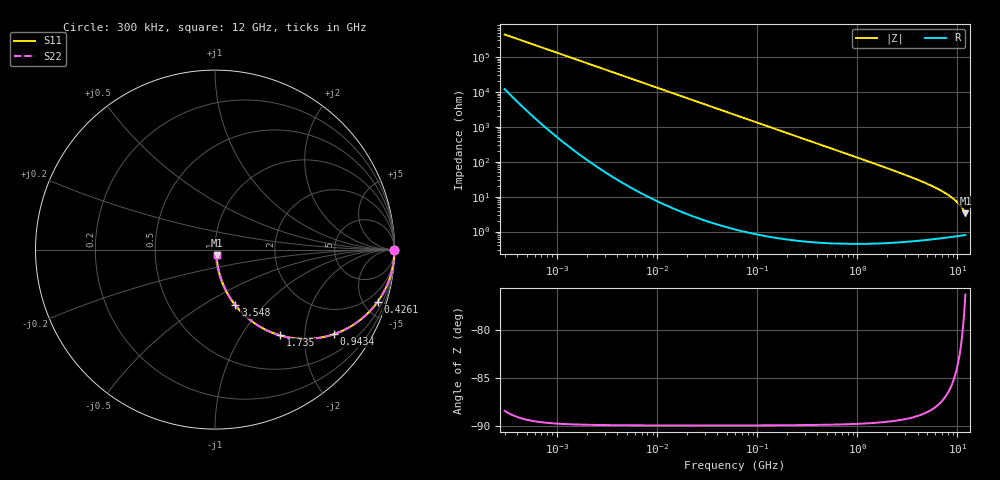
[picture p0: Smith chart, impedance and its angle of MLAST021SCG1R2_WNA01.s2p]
! MLAST021SCG1R2_WNA01  S-PARAMETER MODEL  ( General Type )
! Model Generated by TAIYO YUDEN Corporation (http://www.ty-top.com)
! Version 1.0
! TAIYO YUDEN Control No. 220901
! Copyright(c) 2022 TAIYO YUDEN CO.,LTD. All Rights Reserved.
! Product Description (link to TY-COMPAS)
! https://ds.yuden.co.jp/TYCOMPAS/or/detail?pn=MLAST021SCG1R2BWNA01&u=M
! Products Name : Multilayer Ceramic Capacitors
! Characteristics :
!  Capacitance : 1.2 pF , Rated Voltage : 25V , TCC : CG / C0G
!  Case Size : 0.25 x 0.125 / 0.0098 x 0.0049 [mm/inch] , Thickness : 0.125 / 0.0049 [mm/inch]
!  (Conditions: Temperature = 25 degC , DC Bias Current/Voltage = 0A / 0V)
! External Node Assignments :
!  1  o---| |---o  2
! GND o---------o GND
! Frequency Range : 0.3MHz  -  12000MHz  [ 401 STEP ]
# MHz S RI R 50
! Freq[MHz].  S11 Real  S11 Imag  S21 Real  S21 Imag  S12 Real  S12 Imag  S22 Real  S22 Imag
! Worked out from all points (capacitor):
!   401 points, 300 kHz to 12 GHz, reference 50 ohm
!   read as one part in series: C = 1.2 pF near 316.3 kHz
!   lowest |Z| = 3.38 ohm at 12 GHz (marker M1)
!   S11 on the Smith chart (normalised r, x): 300 kHz: open; 426.1 MHz: 1.01, -6.22; 943.4 MHz: 1.01, -2.80; 1.735 GHz: 1.01, -1.51; 3.548 GHz: 1.01, -0.70; 12 GHz: 1.02, -0.07
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0.3  1 -0.000226  6.2e-06 0.000226  6.2e-06 0.000226  1 -0.000226
1.769972  1 -0.00133  4.34e-06 0.00133  4.34e-06 0.00133  1 -0.00133
10.44266  0.9999 -0.00787  6.63e-05 0.00787  6.63e-05 0.00787  0.9999 -0.00787
60  0.9979 -0.0451  0.00207 0.0451  0.00207 0.0451  0.9979 -0.0451
159.8975  0.9856 -0.1188  0.0144 0.1188  0.0144 0.1188  0.9856 -0.1188
237.9135  0.9686 -0.1738  0.0314 0.1738  0.0314 0.1738  0.9686 -0.1738
353.9943  0.9331 -0.2491  0.0669 0.2491  0.0669 0.2491  0.9331 -0.2491
426.1204  0.9059 -0.2912  0.0941 0.2912  0.0941 0.2912  0.9059 -0.2912
634.0297  0.8129 -0.3889  0.1871 0.3889  0.1871 0.3889  0.8129 -0.3889
943.3804  0.6616 -0.4716  0.3384 0.4716  0.3384 0.4716  0.6616 -0.4716
1296.429  0.5072 -0.4977  0.4928 0.4977  0.4928 0.4977  0.5072 -0.4977
1735.023  0.3628 -0.4778  0.6372 0.4778  0.6372 0.4778  0.3628 -0.4778
2088.533  0.2801 -0.4453  0.7199 0.4453  0.7199 0.4453  0.2801 -0.4453
2722.03  0.1833 -0.3817  0.8167 0.3817  0.8167 0.3817  0.1833 -0.3817
3547.679  0.1132 -0.3095  0.8868 0.3095  0.8868 0.3095  0.1132 -0.3095
5565.855  0.0445 -0.1921  0.9555 0.1921  0.9555 0.1921  0.0445 -0.1921
6699.894  0.0292 -0.1491  0.9708 0.1491  0.9708 0.1491  0.0292 -0.1491
7854.144  0.0201 -0.1148  0.9799 0.1148  0.9799 0.1148  0.0201 -0.1148
9708.23  0.0125 -0.0722  0.9875 0.0722  0.9875 0.0722  0.0125 -0.0722
10511.28  0.0108 -0.057  0.9892 0.057  0.9892 0.057  0.0108 -0.057
11380.75  0.00953 -0.042  0.9905 0.042  0.9905 0.042  0.00953 -0.042
12000  0.00897 -0.0322  0.991 0.0322  0.991 0.0322  0.00897 -0.0322
